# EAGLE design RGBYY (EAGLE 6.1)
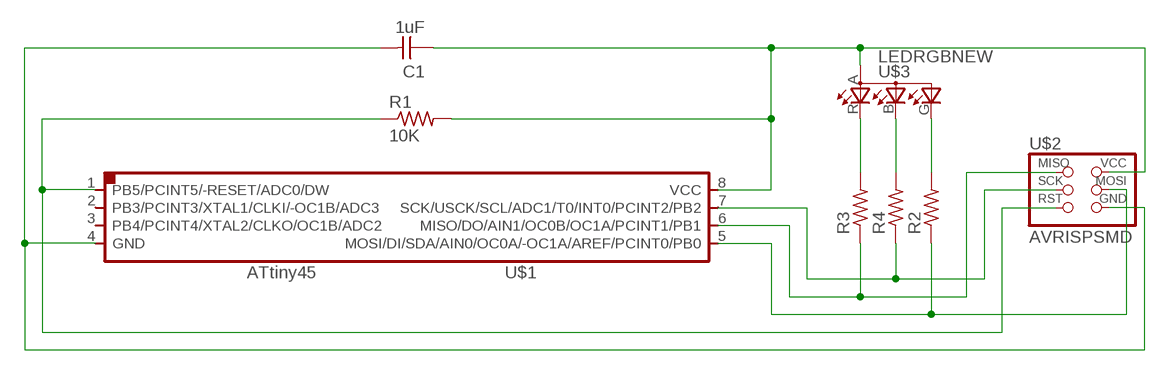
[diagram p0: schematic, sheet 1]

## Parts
C1  1uF  CAP-UNPOLARIZEDFAB  [C1206FAB]
R1  10K  RES-US1206FAB  [R1206FAB]
R2  RES-US1206FAB  [R1206FAB]
R3  RES-US1206FAB  [R1206FAB]
R4  RES-US1206FAB  [R1206FAB]
U$1  ATTINY45SI  [SOIC8]
U$2  AVRISPSMD  [2X03SMD]
U$3  LEDRGBNEW  [P-LCC-4]

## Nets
N$1: C1.2 U$1.4(GND) U$2.6(GND)
N$2: C1.1 R1.2 U$1.8(VCC) U$2.2(VCC) U$3.A(A2)
N$3: R3.2 U$3.R(CRED)
N$4: R4.2 U$3.B(CBLUE)
N$5: R2.2 U$3.G(CGREEN)
N$6: R4.1 U$1.7(SCK/USCK/SCL/ADC1/T0/INT0/PCINT2/PB2) U$2.3(SCK)
N$7: R3.1 U$1.6(MISO/DO/AIN1/OC0B/OC1A/PCINT1/PB1) U$2.1(MISO)
N$8: R2.1 U$1.5(MOSI/DI/SDA/AIN0/OC0A/-OC1A/AREF/PCINT0/PB0) U$2.4(MOSI)
N$9: R1.1 U$1.1(PB5/PCINT5/-RESET/ADC0/DW) U$2.5(RST)
Unconnected: U$1.2(PB3/PCINT3/XTAL1/CLKI/-OC1B/ADC3) U$1.3(PB4/PCINT4/XTAL2/CLKO/OC1B/ADC2)

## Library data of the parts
C1 = fab:CAP-UNPOLARIZED
R1-R4 = fab:RES-US: Resistor (US Symbol)
U$1 = fab:ATTINY45
U$2 = fab:AVRISP
U$3 = fab:LEDRGBNEW

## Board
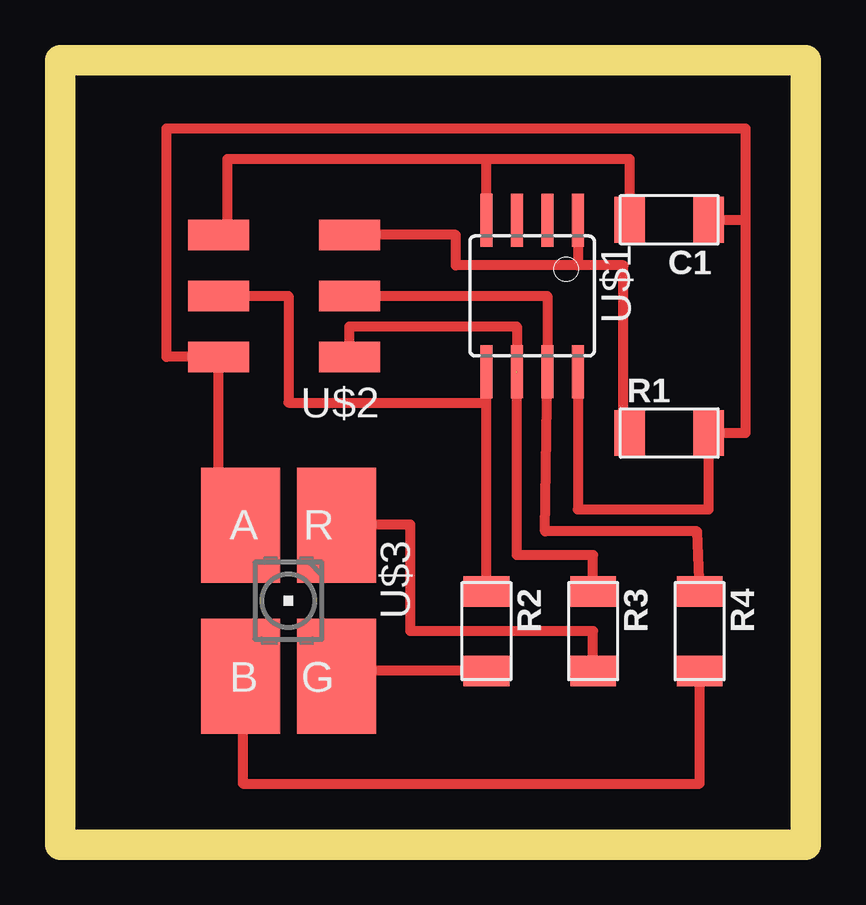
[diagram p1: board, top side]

Size 31.09 x 32.69 mm. Coordinates in mm from the lower left corner, seen from the top.
Outline: 0,0 31.09,0 31.09,32.69 0,32.69 0,0
Copper layers (1*16): Top 0.035mm / dielectric 1.5mm / Bottom 0.035mm
Design rules: minimum track width 10mil, minimum drill 24mil, track to track 8mil, track to pad 8mil, pad to pad 8mil, via to via 8mil, smd to smd 8mil, copper to edge 40mil, drill to drill 8mil, minimum pad ring 10mil, minimum via ring 8mil, stop-mask expansion 4mil, vias tented up to drill 0mil, thermal gap 10mil

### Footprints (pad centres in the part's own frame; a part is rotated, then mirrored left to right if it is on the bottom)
C1206FAB = smd 1.27 x 1.905: 1 -1.651,0; 2 1.651,0
R1206FAB = smd 1.27 x 1.905: 1 -1.651,0; 2 1.651,0
SOIC8 = smd 0.5 x 2.2: 1 -1.905,-3.154; 2 -0.645,-3.154; 3 0.625,-3.154; 4 1.895,-3.154; 5 1.905,3.154; 6 0.635,3.154; 7 -0.635,3.154; 8 -1.905,3.154
2X03SMD = smd 2.54 x 1.27: 1 -2.54,2.54; 2 2.92,2.54; 3 -2.54,0; 4 2.92,0; 5 -2.54,-2.54; 6 2.92,-2.54
P-LCC-4 = smd 3.3 x 4.8: A 2,-3.15; B 2,3.15; G -2,3.15; R -2,-3.15

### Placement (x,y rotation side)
C1  25.4,26.04 180 top
R1  25.4,17.15 0 top
R2  17.78,8.89 270 top
R3  22.23,8.89 270 top
R4  26.67,8.89 270 top
U$1  19.68,22.86 180 top
U$2  9.53,22.86 180 top
U$3  9.53,10.16 180 top

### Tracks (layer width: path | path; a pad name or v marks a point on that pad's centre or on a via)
N$1
  Top 0.406: U$2.6 6.99,25.4 6.99,28.58 17.78,28.58 | 17.78,28.58 23.75,28.58 C1.2 | U$1.4 17.78,28.58
N$2
  Top 0.406: U$3.A 6.61,13.31 U$2.2 4.45,20.32 4.45,29.85 28.57,29.85 28.57,26.04 | U$1.8 21.59,13.97 27.05,13.97 R1.2 28.57,17.15 28.57,26.04 | C1.1 28.57,26.04
N$3
  Top 0.406: R3.2 22.23,8.89 14.61,8.89 14.61,13.33 11.53,13.33 U$3.R
N$4
  Top 0.406: U$3.B 7.62,7.01 7.62,2.54 26.67,2.54 R4.2
N$5
  Top 0.406: R2.2 11.53,7.24 U$3.G
N$6
  Top 0.406: R4.1 26.57,13.05 20.22,13.05 U$1.7 20.32,22.86 U$2.3
N$7  (1 unrouted)
  Top 0.406: R3.1 22.23,12.06 19.05,12.06 19.05,19.69 U$1.6 19.05,21.59 12.06,21.59 U$2.1
N$8
  Top 0.406: R2.1 17.78,18.42 | 17.78,18.42 U$1.5 | U$2.4 9.53,22.86 9.53,18.42 17.78,18.42
N$9
  Top 0.406: U$1.1 21.59,24.13 | 21.59,24.13 16.51,24.13 16.51,25.4 U$2.5 | R1.1 23.5,17.15 23.5,24.13 21.59,24.13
